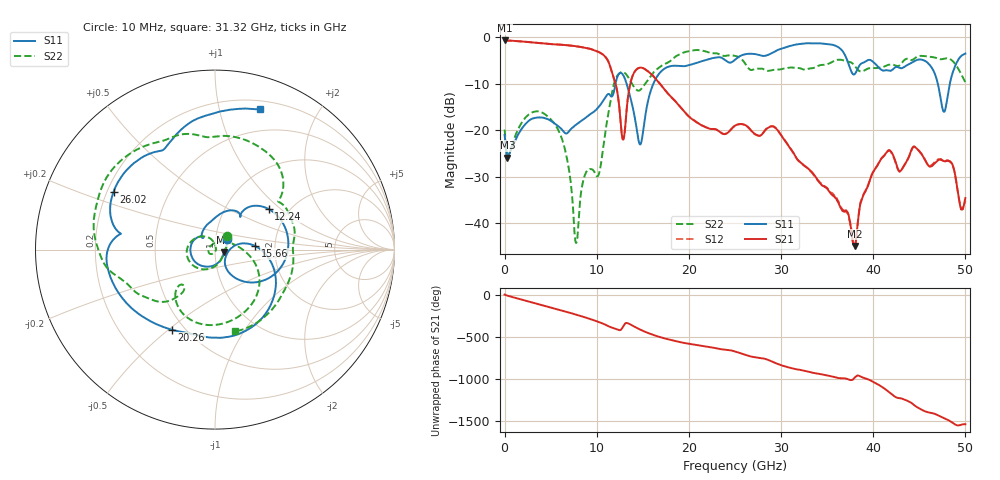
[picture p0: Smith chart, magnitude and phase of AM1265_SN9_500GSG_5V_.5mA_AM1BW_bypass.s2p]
!Keysight Technologies,N5245B,MY58422270,A.16.20.02
!Date: Thursday, March 05, 2026 01:51:12
!Correction: S11(C  2-Port  )
!S21(C  2-Port  )
!S12(C  2-Port  )
!S22(C  2-Port  )
!S2P File: Measurements: S11, S21, S12, S22:
# Hz S  dB  R 50
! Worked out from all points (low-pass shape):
!   3201 points, 10 MHz to 50 GHz, reference 50 ohm
!   highest |S21| = -0.73 dB at 10 MHz (marker M1); lowest = -44.9 dB at 38.02 GHz (marker M2)
!   |S21| within 3 dB of the highest: start of sweep to 10.66 GHz
!   lowest |S11| = -25.9 dB at 306.8 MHz (marker M3), VSWR 1.11, Z = 55.1 - j1.67 ohm
!   |S11| at or under -10 dB: start of sweep to 12.05 GHz; 13.24 GHz to 16.16 GHz (2.914 GHz wide, 19.8 % of centre); 47.01 GHz to 48.31 GHz (1.305 GHz wide, 2.74 % of centre)
!   |S22| runs from -44.2 to -2.8 dB; largest |S21 - S12| = 0.0058
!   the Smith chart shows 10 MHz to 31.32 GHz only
!   S11 on the Smith chart (normalised r, x): 10 MHz: 1.13, +0.14; 12.24 GHz: 1.58, +0.83; 15.66 GHz: 1.58, +0.07; 20.26 GHz: 0.43, -0.52; 26.02 GHz: 0.23, +0.25; 31.32 GHz: 0.28, +1.34
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1e7  -21.01 43.7  -0.73 4.4  -0.76 4.1  -19.86 47.9
3.068156e8  -25.87 -17.3  -0.76 -8.8  -0.76 -8.9  -26.10 -18.3
3.415569e9  -17.31 -167.1  -1.23 -101.8  -1.22 -101.8  -15.95 -163.5
5.961934e9  -19.35 136.9  -1.62 -177.5  -1.62 -177.5  -20.50 128.9
7.727206e9  -18.88 130.3  -1.96 126.7  -1.97 126.6  -44.11 -2.6
8.352081e9  -17.97 121.4  -2.16 105.9  -2.16 105.9  -32.74 -115.9
1.057039e10  -14.09 82.8  -3.61 22.8  -3.61 22.7  -25.72 55.7
1.224193e10  -8.53 37.2  -11.84 -53.0  -11.85 -53.2  -8.27 -65.5
1.288242e10  -8.20 -11.1  -21.97 -13.6  -21.99 -13.8  -7.52 -102.4
1.467894e10  -23.02 -28.3  -6.58 -50.7  -6.58 -50.7  -11.43 -129.8
1.566312e10  -12.93 5.0  -7.51 -97.2  -7.51 -97.3  -8.97 -129.8
1.667854e10  -8.10 -30.5  -9.61 -135.9  -9.60 -136.0  -6.69 -144.5
2.025595e10  -5.90 -118.1  -17.50 133.8  -17.45 133.7  -2.95 155.8
2.5005e10  -4.88 167.7  -19.03 46.4  -19.03 46.5  -4.04 70.2
2.602042e10  -3.73 150.3  -18.82 10.5  -18.81 10.4  -5.45 44.5
3.131624e10  -1.72 72.1  -24.76 -157.0  -24.86 -157.4  -6.56 -76.1
3.334708e10  -1.34 35.6  -28.98 155.5  -29.17 155.6  -6.69 -127.2
3.801802e10  -7.89 -26.4  -44.86 99.0  -44.76 102.5  -6.22 137.5
4.167354e10  -7.19 -56.1  -24.31 -73.8  -24.34 -74.7  -5.95 113.7
4.53603e10  -4.91 -99.6  -25.50 66.9  -25.45 65.8  -4.04 72.6
4.778169e10  -15.79 76.9  -26.65 -31.4  -26.58 -31.4  -4.61 39.7
5e10  -3.55 -70.2  -34.55 -99.4  -35.11 -104.6  -9.72 4.8
